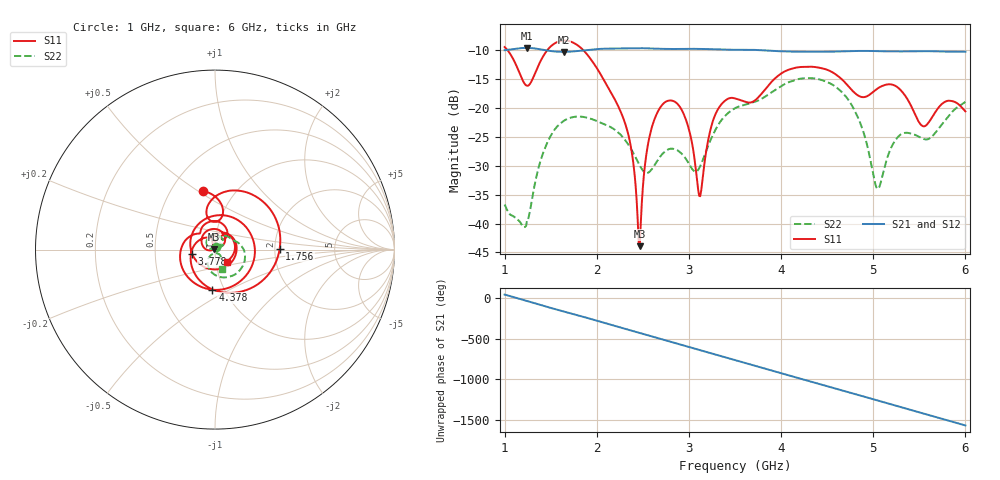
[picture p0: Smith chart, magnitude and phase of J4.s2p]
!Agilent Technologies,E8364B,MY43040528,A.07.50.67
!Agilent E8364B: A.07.50.67
!Date: Sunday, March 01, 2026 18:21:15
!Correction: S11(Full 2 Port(1,2))
!S21(Full 2 Port(1,2))
!S12(Full 2 Port(1,2))
!S22(Full 2 Port(1,2))
!S2P File: Measurements: S11, S21, S12, S22:
# Hz S  dB  R 50
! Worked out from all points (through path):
!   451 points, 1 GHz to 6 GHz, reference 50 ohm
!   highest |S21| = -9.67 dB at 1.244 GHz (marker M1); lowest = -10.4 dB at 1.644 GHz (marker M2)
!   group delay of S21, straight-line fit = 897 ps
!   lowest |S11| = -43.9 dB at 2.467 GHz (marker M3), VSWR 1.01, Z = 49.4 + j0.267 ohm
!   |S11| at or under -10 dB: 1.028 GHz to 1.467 GHz (438.4 MHz wide, 35.1 % of centre); 1.85 GHz to end of sweep
!   |S22| runs from -40.6 to -14.9 dB; largest |S21 - S12| = 0.0015
!   S11 on the Smith chart (normalised r, x): 1 GHz: 0.71, +0.52; 1.756 GHz: 2.13, +0.03; 3.778 GHz: 0.77, -0.04; 4.378 GHz: 0.88, -0.41; 6 GHz: 1.13, -0.15
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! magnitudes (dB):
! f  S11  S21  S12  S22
! 1 GHz  -9.5  -10.1  -10.1  -36.7
! 1.244 GHz  -16.2  -9.7  -9.7  -39.3
! 1.422 GHz  -11.0  -10.0  -10.0  -27.6
! 1.644 GHz  -8.4  -10.4  -10.4  -22.2
! 1.756 GHz  -8.9  -10.3  -10.3  -21.6
! 1.844 GHz  -9.9  -10.1  -10.1  -21.6
! 2.311 GHz  -22.9  -9.8  -9.8  -25.7
! 2.467 GHz  -43.9  -9.7  -9.8  -30.0
! 2.544 GHz  -27.4  -9.7  -9.8  -31.3
! 2.667 GHz  -20.5  -9.8  -9.8  -28.9
! 2.922 GHz  -20.4  -9.8  -9.9  -28.0
! 3.122 GHz  -35.3  -9.8  -9.9  -30.1
! 3.278 GHz  -21.5  -9.9  -10.0  -24.1
! 3.5 GHz  -18.4  -10.0  -10.0  -20.1
! 3.778 GHz  -17.8  -10.1  -10.1  -18.6
! 4.344 GHz  -12.9  -10.3  -10.4  -14.9
! 4.378 GHz  -13.0  -10.3  -10.4  -15.0
! 4.767 GHz  -16.9  -10.2  -10.2  -19.6
! 5.044 GHz  -16.7  -10.2  -10.3  -34.0
! 5.167 GHz  -16.0  -10.3  -10.3  -28.0
! 5.533 GHz  -23.1  -10.2  -10.3  -25.3
! 6 GHz  -20.6  -10.3  -10.4  -19.0
